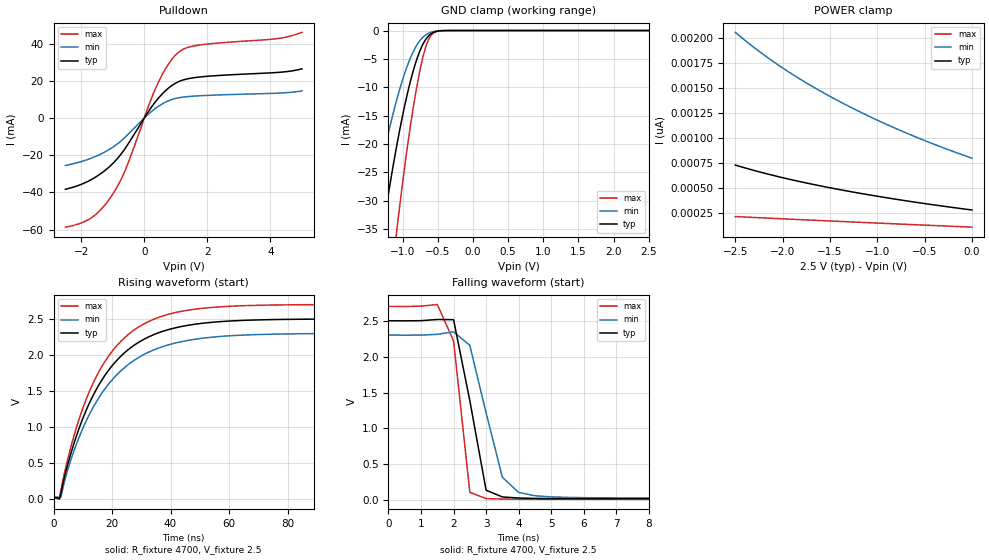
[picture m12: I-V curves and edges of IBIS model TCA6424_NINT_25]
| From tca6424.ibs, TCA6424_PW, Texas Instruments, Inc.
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[Model]   TCA6424_NINT_25
Model_type  Open_drain
Enable   Active-Low
Vref =   2.5
Rref =   4700
Cref =   50p
Vmeas =   1.25
| variable   typ   min   max
C_comp   2.36pF   1.83pF   2.59pF
| C_pulldown   3.31pF   2.36pF   4.14pF
| C_tri-state   2.36pF   1.83pF   2.59pF
[Temperature Range]   40   100   -40
| Ambient temperature   25   85   -40
[Voltage range]   2.5   2.3   2.7
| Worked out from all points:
|   slope of the pulldown table from 0 to 0.375 V, typ, clamps not added: 41 ohm
|   GND clamp passes 1 mA (typ) near -0.63 V on its own axis
|   rising waveform, R_fixture 4700, V_fixture 2.5: 20-80 % time 18.5ns typ, 19.5ns min, 17.6ns max; typ from 0.019 V to 2.5 V
|   falling waveform, R_fixture 4700, V_fixture 2.5: 20-80 % time 623ps typ, 743ps min, 382ps max; typ from 2.5 V to 0.019 V
[GND Clamp]
| TCA6424_NINT_25
|   Voltage   I(typ)   I(min)   I(max)
-2.5V     -162.5mA   -117.5mA   -234.5mA
-1.495V   -53.75mA   -35.77mA   -85.47mA
-1.465V   -51mA      -33.78mA   -81.48mA
-1.275V   -34.61mA   -22.1mA    -57.29mA
-1.085V   -20.46mA   -12.31mA   -35.57mA
-960mV    -12.71mA   -7.198mA   -23.11mA
-840mV    -6.756mA   -3.54mA    -12.99mA
-730mV    -2.913mA   -1.434mA   -5.728mA
-650mV    -1.229mA   -608.9uA   -2.183mA
-575mV    -416.4uA   -230.2uA   -590.2uA
-445mV    -34.41uA   -26.43uA   -31.67uA
2.5V      278.2pA    863.6pA    98.69pA
[POWER Clamp]
| TCA6424_NINT_25
|   Voltage   I(typ)   I(min)   I(max)
-2.5V     727.1pA    2.053nA    212.7pA
-2.25V    660.1pA    1.864nA    201.2pA
-2.005V   602.1pA    1.701nA    190.3pA
-1.705V   539.2pA    1.523nA    177.3pA
-1.405V   483.1pA    1.365nA    164.5pA
-1.095V   430.7pA    1.218nA    151.5pA
-745mV    377.1pA    1.068nA    137pA
-380mV    326.3pA    927.6pA    122.1pA
-31.15fV  278.2pA    796.2pA    106.7pA
[Pulldown]
| TCA6424_NINT_25
|   Voltage   I(typ)   I(min)   I(max)
-2.5V     -38.28mA   -25.48mA   -58.63mA
-1.665V   -32.94mA   -21.48mA   -53.47mA
-1.325V   -29.22mA   -18.91mA   -48.24mA
-1.005V   -24.56mA   -15.75mA   -41.05mA
-585mV    -15.83mA   -9.951mA   -27.3mA
150mV     3.947mA    2.363mA    7.134mA
425mV     10.19mA    6.023mA    18.39mA
760mV     15.97mA    9.213mA    28.81mA
1.09V     19.56mA    10.9mA     35.38mA
1.67V     21.89mA    11.89mA    39.05mA
4.19V     24.47mA    13.35mA    42.64mA
5V        26.46mA    14.57mA    46.07mA
[Ramp]
| TCA6424_NINT_25
| variable   typ   min   max
dV/dt_r   1.50/1.85E-08   1.37/1.95E-08   1.63/1.76E-08
dV/dt_f   1.52/4.48E-10   1.39/6.81E-10   1.64/3.24E-10
R_load = 4700
[Rising Waveform]
| TCA6424_NINT_25
R_fixture =   4700
C_fixture =   0
L_fixture =   0
V_fixture =   2.5
V_fixture_min = 2.3
V_fixture_max = 2.7
|   Time   V(typ)   V(min)   V(max)
0s        19.28mV    29.42mV    11.52mV
2ns       3.79mV     21.48mV    -3.645mV
5ns       500.9mV    424.3mV    578.2mV
9.5ns     1.064V     932.5mV    1.2V
14ns      1.474V     1.305V     1.648V
19.5ns    1.823V     1.629V     2.022V
31.5ns    2.23V      2.018V     2.443V
48.5ns    2.427V     2.219V     2.636V
97ns      2.498V     2.298V     2.699V
520ns     2.5V       2.3V       2.7V
[Falling Waveform]
| TCA6424_NINT_25
R_fixture =   4700
C_fixture =   0
L_fixture =   0
V_fixture =   2.5
V_fixture_min = 2.3
V_fixture_max = 2.7
|   Time   V(typ)   V(min)   V(max)
0s        2.5V       2.3V       2.7V
1.5ns     2.518V     2.311V     2.726V
2ns       2.515V     2.346V     2.22V
2.5ns     1.385V     2.157V     108.8mV
3ns       138.3mV    1.216V     22.09mV
3.5ns     44.82mV    318.6mV    15.68mV
4ns       29.45mV    107.9mV    13.67mV
4.5ns     24.51mV    61.84mV    12.74mV
8.5ns     19.52mV    30.38mV    11.59mV
520ns     19.28mV    29.42mV    11.52mV
